(* Logix 5000 AddOnInstructionDefinition export ACS_INDEXED_MOVE; software revision 20.01 *)

ADD_ON_INSTRUCTION ACS_INDEXED_MOVE   (* revision 2.0, vendor Tolomatic, Inc *)
// Execute a saved indexed move as defined in the drive
VAR_IN_OUT
   DriveMoveSelect : SINT; {required}   // ACS.0.MOVESELECT
END_VAR
VAR_INPUT
   Index : INT; {required}   // Move Index to Execute
END_VAR

ROUTINE Logic   (* ladder *)
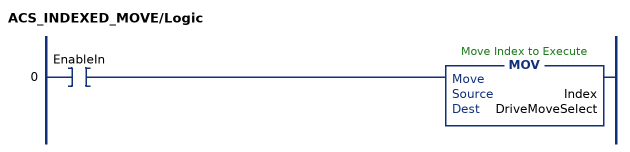
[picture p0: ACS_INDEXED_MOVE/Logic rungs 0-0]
   0: XIC(EnableIn)MOV(Index,DriveMoveSelect);
END_ROUTINE
END_ADD_ON_INSTRUCTION
